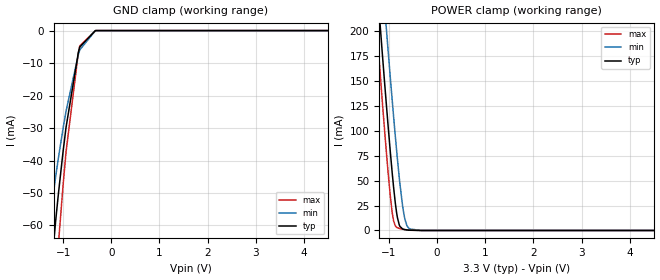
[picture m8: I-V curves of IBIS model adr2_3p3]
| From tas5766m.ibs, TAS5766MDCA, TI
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|   adr2_3p3 Model
[Model]   adr2_3p3
Model_type   Input
Vinl = 0.8
Vinh = 2
|   typ   min   max
|   (nom PVT)   (fast PVT)   (slow PVT)
C_comp   6.093e-12   5.975e-12   6.153e-12
| Where nom  PVT is Nominal Process, 3.3V, 27C
|   Fast PVT is Strong Process,  3.6V, -40C
|   Slow PVT is Weak Process,   3V, 125C
[Voltage Range]   3.3   3   3.6
|Junction Temperature
[Temperature Range]   27   125   -40
[Power Clamp Reference]   3.3   3   3.6
[GND Clamp Reference]   0   0   0
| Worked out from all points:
|   POWER clamp passes 1 mA (typ) near -0.68 V on its own axis
[GND Clamp]
|   Voltage   I(typ)   I(min)   I(max)
-3.3V     -1.431A    -1.15A     -1.715A
-1.383V   -96.16mA   -70.4mA    -129.9mA
-1.154V   -58.38mA   -44.81mA   -77.05mA
-1.097V   -49.99mA   -39.02mA   -65.35mA
-999.9mV  -37.02mA   -29.96mA   -47.34mA
-940.5mV  -29.83mA   -24.86mA   -37.43mA
-684mV    -6.73mA    -7.376mA   -6.767mA
-654mV    -5.034mA   -5.917mA   -4.726mA
-330mV    -4.08uA    -36.46uA   -660.2nA
6.6V      0A         0A         0A
[POWER Clamp]
|   Voltage   I(typ)   I(min)   I(max)
-3.3V     1.645A     1.695A     1.627A
-1.27V    261.1mA    337mA      213.9mA
-1.136V   176.4mA    252.8mA    128.3mA
-1.08V    141.8mA    218.1mA    93.87mA
-1.018V   104.7mA    180.3mA    57.92mA
-934.8mV  58.79mA    131.8mA    18.74mA
-902.4mV  42.66mA    113.4mA    9.456mA
-825mV    13.04mA    71.96mA    2.758mA
-772.8mV  4.126mA    46.94mA    1.891mA
-690mV    1.091mA    16.47mA    1.001mA
-576mV    306.2uA    1.521mA    243.7uA
6.6V      0A         0A         0A
